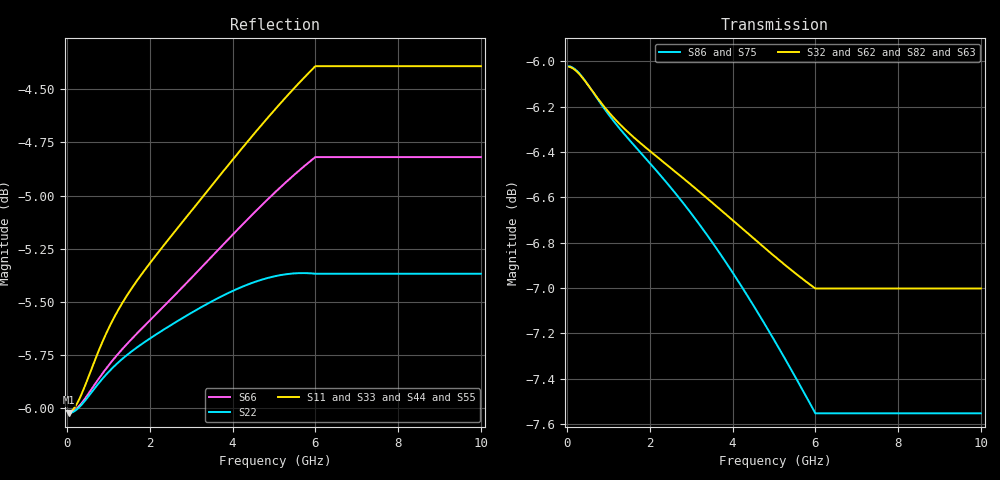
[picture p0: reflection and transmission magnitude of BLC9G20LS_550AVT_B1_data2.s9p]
! Created Tue Aug  4 23:39:32 2015
# ghz S ma R 50
! 9 Port Network Data from SP1.SP block
! freq  magS11  angS11  magS12  angS12  magS13  angS13  magS14  angS14
!  magS15  angS15  magS16  angS16  magS17  angS17  magS18  angS18
!  magS19  angS19
!  magS21  angS21  magS22  angS22  magS23  angS23
!  magS24  angS24  magS25  angS25  magS26  angS26  magS27  angS27
!  magS28  angS28  magS29  angS29
!  magS31  angS31  magS32  angS32
!  magS33  angS33  magS34  angS34  magS35  angS35  magS36  angS36
!  magS37  angS37  magS38  angS38  magS39  angS39
!  magS41  angS41
!  magS42  angS42  magS43  angS43  magS44  angS44  magS45  angS45
!  magS46  angS46  magS47  angS47  magS48  angS48  magS49  angS49
!  magS51  angS51  magS52  angS52  magS53  angS53  magS54  angS54
!  magS55  angS55  magS56  angS56  magS57  angS57  magS58  angS58
!  magS59  angS59
!  magS61  angS61  magS62  angS62  magS63  angS63
!  magS64  angS64  magS65  angS65  magS66  angS66  magS67  angS67
!  magS68  angS68  magS69  angS69
!  magS71  angS71  magS72  angS72
!  magS73  angS73  magS74  angS74  magS75  angS75  magS76  angS76
!  magS77  angS77  magS78  angS78  magS79  angS79
!  magS81  angS81
!  magS82  angS82  magS83  angS83  magS84  angS84  magS85  angS85
!  magS86  angS86  magS87  angS87  magS88  angS88  magS89  angS89
!  magS91  angS91  magS92  angS92  magS93  angS93  magS94  angS94
!  magS95  angS95  magS96  angS96  magS97  angS97  magS98  angS98
!  magS99  angS99
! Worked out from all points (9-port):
!   200 points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, 50 MHz to 10 GHz, reference 50 ohm
!   strongest paths, dB at 50 MHz, 2.55 GHz, 5.05 GHz, 7.55 GHz, 10 GHz:
!     S32: -6.0, -6.5, -6.9, -7.0, -7.0
!     S62: -6.0, -6.5, -6.9, -7.1, -7.1
!     S82: -6.0, -6.5, -6.9, -7.1, -7.1
!     S63: -6.0, -6.5, -7.1, -7.4, -7.4
!     S86: -6.0, -6.6, -7.2, -7.6, -7.6
!     S75: -6.0, -6.8, -7.3, -7.4, -7.4
!   lowest |S11| = -6.0 dB at 50 MHz (marker M1), VSWR 3.00, Z = 16.7 - j0.121 ohm
!   |S11| at or under -10 dB: nowhere
